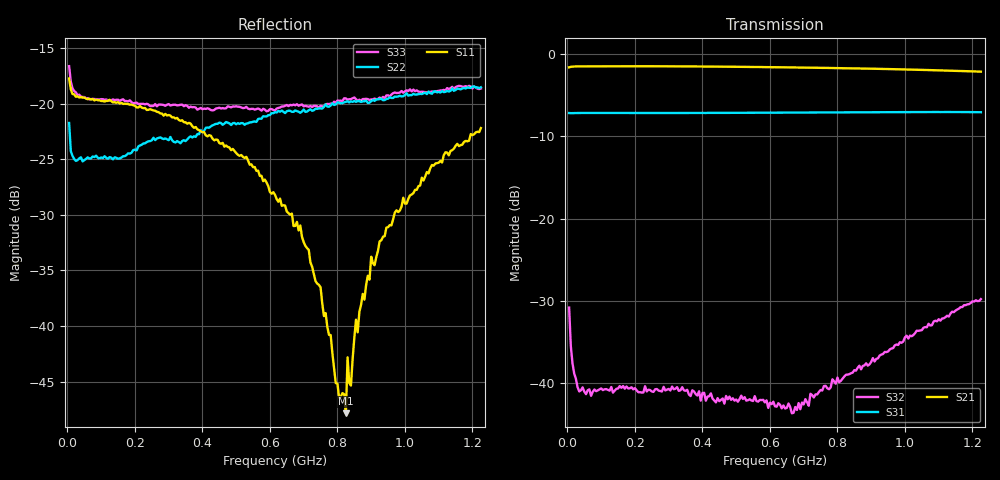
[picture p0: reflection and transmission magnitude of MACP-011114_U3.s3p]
!Agilent Technologies,E5071C,MY46110647,A.11.31
!Date: Tue Jan 09 15:01:13 2024 DD
!Data & Calibration Information:
!MACP-011114 soldered onto PT-0030145 with F connectors, calibration PCB PT-0003653. Port1 (pin1) Port2 (pin6) Port3 (pin3)
!Freq	S11:SOLT3(ON)	S12:SOLT3(ON)	S13:SOLT3(ON)
!	S21:SOLT3(ON)	S22:SOLT3(ON)	S23:SOLT3(ON)
!	S31:SOLT3(ON)	S32:SOLT3(ON)	S33:SOLT3(ON)
!PortZ  Port1:75+j0  Port2:75+j0  Port3:75+j0
!Above PortZ is port z conversion or system Z0 setting when saving the data.
!When reading, reference impedance value at option line is always used.
# Hz S MA R 75
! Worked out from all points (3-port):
!   245 points, 5 MHz to 1.225 GHz, reference 75 ohm
!   strongest paths, dB at 5 MHz, 310 MHz, 615 MHz, 920 MHz, 1.225 GHz:
!     S21: -1.6, -1.5, -1.6, -1.8, -2.1
!     S31: -7.2, -7.2, -7.1, -7.1, -7.1
!     S32: -30.8, -40.4, -42.8, -37.0, -29.8
!   lowest |S11| = -47.9 dB at 825 MHz (marker M1), VSWR 1.01, Z = 74.6 - j0.456 ohm
!   |S11| at or under -10 dB: start of sweep to end of sweep
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5000000  0.1296 158.4  0.8329 3.0  0.4368 -178.7
         0.831 3.1  0.08175 66.1  0.02573 95.7
         0.4382 -178.7  0.02878 97.1  0.1472 151.3
1.5e7  0.1103 169.5  0.8397 0.6  0.4381 179.3
       0.8395 0.6  0.05814 30.4  0.01322 66.5
       0.4378 179.3  0.01318 70.1  0.117 163.3
3.5e7  0.1065 173.4  0.8429 -0.9  0.4387 177.0
       0.8423 -1.0  0.05665 11.9  0.0094 40.9
       0.4388 177.0  0.0089 40.5  0.1096 168.3
6.15e8  0.03885 149.1  0.8316 -29.2  0.441 122.0
        0.8327 -29.1  0.0914 -53.9  0.005877 39.6
        0.4402 122.0  0.007221 46.5  0.09302 106.1
7.15e8  0.02199 149.5  0.8265 -34.1  0.4423 112.6
        0.8276 -34.0  0.09327 -57.2  0.007046 66.3
        0.4417 112.5  0.00728 59.0  0.09667 95.8
8.25e8  0.004046 -131.0  0.8194 -39.5  0.4436 102.2
        0.8207 -39.4  0.1017 -62.8  0.009722 81.0
        0.4424 102.2  0.01123 76.5  0.1054 79.8
8.3e8  0.007219 -130.0  0.8193 -39.7  0.4433 101.7
       0.8199 -39.6  0.1023 -62.6  0.01006 84.7
       0.4425 101.7  0.01126 77.1  0.104 78.8
8.4e8  0.005393 -97.2  0.8183 -40.2  0.4434 100.8
       0.8196 -40.1  0.1023 -63.2  0.01046 84.0
       0.4431 100.7  0.01147 77.5  0.1047 78.7
9e8  0.02047 -86.4  0.8141 -43.2  0.4441 95.1
     0.8152 -43.1  0.1024 -65.2  0.01343 85.1
     0.4438 95.1  0.01344 80.3  0.1043 71.9
1.225e9  0.07754 -93.8  0.7822 -60.0  0.4446 63.5
         0.7823 -59.9  0.1183 -84.3  0.03118 73.4
         0.4433 63.6  0.0324 72.7  0.1168 38.8
